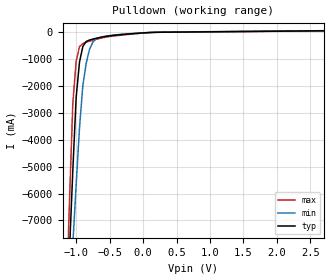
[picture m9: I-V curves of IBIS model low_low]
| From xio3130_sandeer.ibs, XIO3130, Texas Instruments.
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[Model] low_low
Model_type Open_drain
Polarity Non-Inverting
Cref = 2.0pF
Rref = 50
Vref = 1.0V
Vmeas =1.0V
|   typ   min   max
C_comp   1.603pF   1.594pF   1.637pF
[Temperature Range]   25   125   -40
[Voltage Range] 1.50V 1.35V 1.65V
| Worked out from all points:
|   slope of the pulldown table from 0 to 0.225 V, typ, clamps not added: 9.83 ohm
| (Process strength) nominal weak strong
[Pulldown]
-1.5V     -32.22A    -27.92A    -37.5A
-1.15V    -11.15A    -12.34A    -10.21A
-1.1V     -8.142A    -10.12A    -6.307A
-1.05V    -5.146A    -7.892A    -2.656A
-1V       -2.424A    -5.674A    -1.084A
-950mV    -1.112A    -3.561A    -542.3mA
-900mV    -534mA     -1.978A    -423.8mA
-850mV    -350.2mA   -1.158A    -379.4mA
-800mV    -295.8mA   -638.6mA   -341mA
-700mV    -232.8mA   -249.2mA   -271mA
-600mV    -181.4mA   -172.4mA   -210.6mA
3V        54.01mA    56.7mA     51.47mA
[Ramp]
| variable   typ   min   max
dV/dt_r 0.24618V/0.0415301ns  0.25194V/0.0445372ns  0.243V/0.0389342ns
dV/dt_f 0.23754V/0.0399045ns  0.23268V/0.0376058ns  0.2367V/0.0389008ns
R_load = 50
